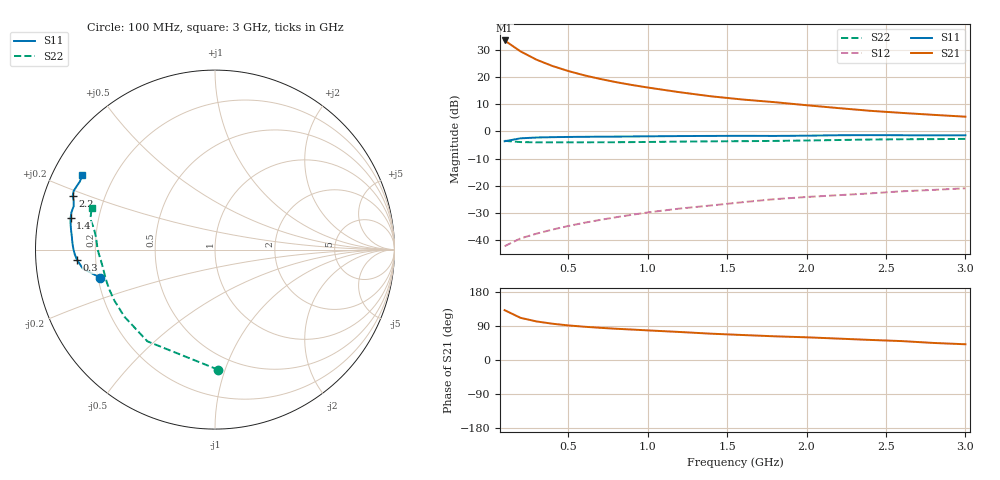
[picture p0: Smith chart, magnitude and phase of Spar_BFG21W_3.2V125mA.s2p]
! Filename: 3_2125bfg21.001
! Title: BFG21W
! Bias: Vce=3.2V; Ic=125mA
! Company: NXP Semiconductors NL
! User: Quality&Reliability T&D
! Measure time: 10 Nov 1999 / 11:43:06
#  MHz  S  MA  R 50
! Freq  S11  S21  S12  S22  :
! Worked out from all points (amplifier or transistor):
!   20 points, 100 MHz to 3 GHz, reference 50 ohm
!   highest |S21| = 33.4 dB at 100 MHz (marker M1)
!   |S21| within 3 dB of that: start of sweep to 174.9 MHz
!   unconditionally stable (mu >= 1): 637 MHz to end of sweep
!   at 400 MHz: K = 0.90, MSG = 30.0 dB, |S12| = -36.1 dB
!   at 1.2 GHz: K = 1.06, MAG = 19.9 dB, |S12| = -28.4 dB
!   at 3 GHz: K = 1.05, MAG = 11.8 dB, |S12| = -20.9 dB
!   S11 on the Smith chart (normalised r, x): 100 MHz: 0.21, -0.12; 300 MHz: 0.13, -0.04; 1.4 GHz: 0.10, +0.11; 2.2 GHz: 0.09, +0.18; 3 GHz: 0.09, +0.26
100  0.6575 -166.2  46.57 131.5  0.007802 57.6  0.6698 -88.4
200  0.7439 -171.8  29.37 111.3  0.01083 54.4  0.635 -126.4
300  0.7698 -175.6  20.71 101.8  0.01322 57.3  0.628 -143.5
400  0.7819 -178.1  15.86 95.8  0.0157 60.9  0.6284 -153.1
500  0.7888 179.8  12.81 91.3  0.01829 63.8  0.6292 -159.2
600  0.7933 178.1  10.69 87.8  0.02093 65.9  0.6298 -163.5
700  0.7973 176.4  9.177 85.0  0.02364 67.7  0.6302 -166.9
800  0.8005 174.9  8.009 82.5  0.02647 69.2  0.6314 -169.7
900  0.805 173.5  7.103 80.4  0.02937 70.7  0.6343 -172.1
1000  0.8101 172.1  6.377 78.2  0.03245 71.4  0.6379 -174.3
1200  0.8184 169.6  5.231 74.0  0.03818 72.2  0.6473 -177.8
1400  0.8238 167.6  4.391 69.4  0.04364 72.5  0.6554 179.3
1600  0.8262 165.3  3.832 65.9  0.05008 72.6  0.6597 176.7
1800  0.8237 163.0  3.428 62.5  0.05692 72.6  0.6672 174.0
2000  0.832 161.1  3.015 59.9  0.06234 73.0  0.6788 171.3
2200  0.8479 159.2  2.672 56.5  0.06729 72.7  0.693 169.0
2400  0.8525 157.4  2.381 53.0  0.07256 71.8  0.707 167.3
2600  0.8482 155.6  2.179 49.9  0.07928 70.7  0.7157 165.7
2800  0.843 153.3  2.007 45.0  0.08423 68.9  0.7196 163.7
3000  0.8473 150.8  1.857 41.5  0.0901 67.9  0.7264 161.2
